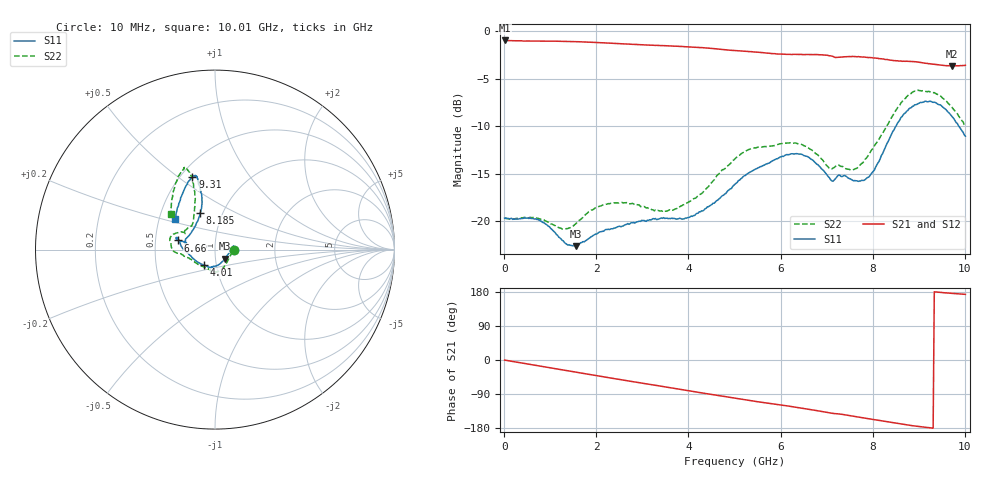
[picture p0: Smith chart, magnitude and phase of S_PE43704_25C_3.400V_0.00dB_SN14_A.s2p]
! Device ID: PE43704
! Dir: z:\PE43704\PE43704_Char_1_20130516\PE43704\AMB\3p400V\0p00dB
! Serial: 14
! Insertion: A
! Impedance: 50 ohm
! Temp: Amb
! VDD: 3.400V
! Attenuation Step: 0.00dB
! IDD: 1.141682e-01mA
#  Hz  S  RI  R  50
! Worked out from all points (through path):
!   401 points, 10 MHz to 10.01 GHz, reference 50 ohm
!   highest |S21| = -0.99 dB at 10 MHz (marker M1); lowest = -3.7 dB at 9.71 GHz (marker M2)
!   group delay of S21, straight-line fit = 53.2 ps
!   lowest |S11| = -22.6 dB at 1.56 GHz (marker M3), VSWR 1.16, Z = 55.4 - j5.68 ohm
!   |S11| at or under -10 dB: start of sweep to 8.502 GHz; 9.867 GHz to end of sweep
!   |S22| runs from -20.8 to -6.2 dB; largest |S21 - S12| = 0.0059
!   S11 on the Smith chart (normalised r, x): 10 MHz: 1.23, +0.00; 4.01 GHz: 0.87, -0.15; 6.66 GHz: 0.66, +0.07; 8.185 GHz: 0.78, +0.34; 9.31 GHz: 0.57, +0.56; 10.01 GHz: 0.60, +0.22
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1e7  0.1041 0.000153  0.8923 -0.00383  0.8925 -0.00349  0.1037 0.000162
7.35e8  0.1009 0.0171  0.8548 -0.2308  0.8548 -0.2305  0.1033 0.0101
1.285e9  0.0754 -0.0233  0.7901 -0.3933  0.79 -0.3931  0.0826 -0.039
1.56e9  0.0538 -0.051  0.7445 -0.468  0.7443 -0.4681  0.0654 -0.0722
1.685e9  0.0445 -0.0634  0.7209 -0.5005  0.7208 -0.5004  0.0555 -0.0875
2.36e9  0.000817 -0.0916  0.5713 -0.6453  0.5717 -0.6452  0.00738 -0.1242
3.36e9  -0.0265 -0.0995  0.3111 -0.78  0.3119 -0.7797  -0.039 -0.1069
4.01e9  -0.0597 -0.0864  0.126 -0.815  0.1267 -0.8154  -0.0984 -0.0794
5.01e9  -0.1561 -0.0165  -0.1478 -0.776  -0.1475 -0.7763  -0.2126 -0.0193
5.335e9  -0.1812 0.00853  -0.2272 -0.7462  -0.227 -0.7462  -0.2396 0.00277
6.085e9  -0.2112 0.0672  -0.3797 -0.6533  -0.3771 -0.6522  -0.2521 0.0544
6.66e9  -0.2059 0.0511  -0.4948 -0.5676  -0.4958 -0.5658  -0.2204 0.0908
6.685e9  -0.2047 0.0513  -0.4999 -0.5628  -0.5004 -0.5616  -0.218 0.0913
7.11e9  -0.159 0.0376  -0.5689 -0.4706  -0.5702 -0.4717  -0.1668 0.0885
7.585e9  -0.1426 0.0795  -0.6267 -0.3839  -0.6259 -0.3829  -0.1276 0.1371
7.885e9  -0.1138 0.1264  -0.6568 -0.3118  -0.6566 -0.3149  -0.1184 0.1843
8.185e9  -0.0823 0.2058  -0.6733 -0.2411  -0.6715 -0.2441  -0.1122 0.2611
8.36e9  -0.0724 0.2614  -0.6761 -0.1972  -0.6757 -0.2008  -0.1127 0.3157
8.835e9  -0.0949 0.3844  -0.6872 -0.0845  -0.6836 -0.0861  -0.1537 0.4442
9.31e9  -0.1262 0.4028  -0.6699 -0.00248  -0.6699 5.18e-05  -0.1817 0.4388
9.71e9  -0.1817 0.3087  -0.6541 0.0492  -0.6516 0.0506  -0.2312 0.3276
1.001e10  -0.223 0.1699  -0.6563 0.0778  -0.6594 0.0783  -0.2466 0.2004
